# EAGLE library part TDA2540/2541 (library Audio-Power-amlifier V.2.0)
The TDA2540 and 2541 are IF amplifier and A.M. demodulator circuits for colour and black and white televisionreceiversusingPNPorNPNtuners. They are intended for reception of negative or positive modulation CCIR standard.
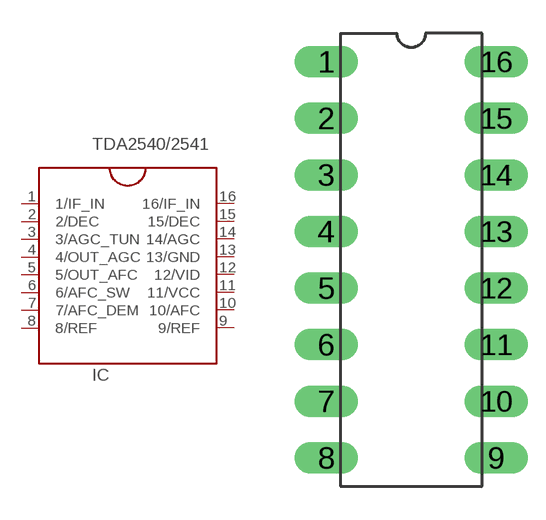
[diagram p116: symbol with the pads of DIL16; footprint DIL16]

Designator prefix IC

## TDA2540/2541  [DIL16]
1  1/IF_IN  in
2  2/DEC
3  3/AGC_TUN
4  4/OUT_AGC  out
5  5/OUT_AFC  out
6  6/AFC_SW
7  7/AFC_DEM
8  8/REF
9  9/REF
10  10/AFC
11  11/VCC  pwr
12  12/VID  out
13  13/GND  pwr
14  14/AGC
15  15/DEC
16  16/IF_IN  in

## Footprint DIL16 (pad centres in mm)
drill 0.8 pad 1.422 long: 1 -3.81,8.89; 2 -3.81,6.35; 3 -3.81,3.81; 4 -3.81,1.27; 5 -3.81,-1.27; 6 -3.81,-3.81; 7 -3.81,-6.35; 8 -3.81,-8.89; 9 3.81,-8.89; 10 3.81,-6.35; 11 3.81,-3.81; 12 3.81,-1.27; 13 3.81,1.27; 14 3.81,3.81; 15 3.81,6.35; 16 3.81,8.89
